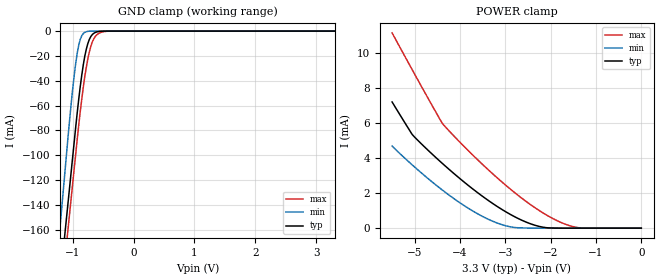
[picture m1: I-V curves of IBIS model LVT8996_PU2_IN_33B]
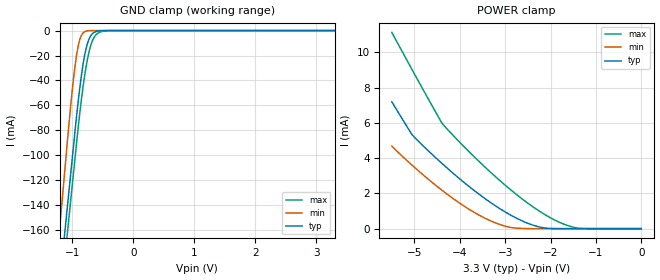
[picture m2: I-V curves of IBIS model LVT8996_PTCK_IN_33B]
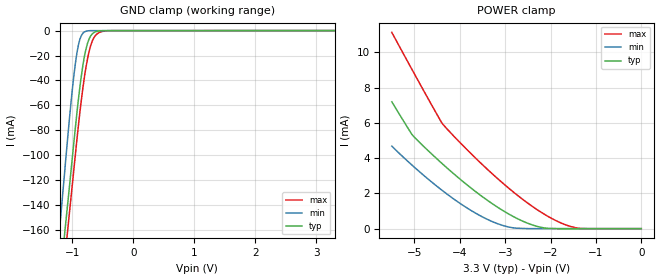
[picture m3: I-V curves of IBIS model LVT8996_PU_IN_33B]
| TEXAS INSTRUMENTS INCORPORATED
| Standard Linear and Logic Group
| IBIS Model of SN74LVT8996
| 3.3-V 10-BIT ADDRESSABLE SCAN PORTS
| This file contains package information for the following:
|  SOIC 24-pin (DW) package as [Component] IBIS_TOP_DW
| This device can be powered at the following Vccs:
|  3.3 volt Vcc
| This file provides unique models under the [Model Selector] for each Vcc.
| For operation at a specific Vcc, select the appropriate model after each
| [Model Selector] keyword.
[IBIS Ver]   3.2
[Comment char]  |_char
[File Name]   sn74lvt8996.ibs
[File Rev]   1.1 | x_die
[Date]   Apr 2, 2004
[Source]   Data created from TI-SPICE simulations at TI-SLL.
[Notes]   The following is an IBIS list for the IBIS_TOP.
   Please contact sllibis@ti.com with questions and
   comments concerning SLL IBIS models.
   NOTE:  The gnd_clamp, pwr_clamp, pullup, and pulldown data
   for ranges beyond GND-VCC may have modeling inaccuracies due
   to convergence problems over the extended IBIS ranges.
|   FILE REV HISTORY
|   1.1  Package R,L C data corrected.
[Disclaimer] Property of Texas Instruments Incorporated.  Unauthorized
   reproduction and/or distribution is strictly prohibited.
   This product is protected under copyright law.
   Created  2002, (C) Copyright  2002, Texas Instruments
   Incorporated, All Rights Reserved
   UNLESS THERE IS A SIGNED, WRITTEN AGREEMENT TO THE
   CONTRARY, TEXAS INSTRUMENTS (TI) IS PROVIDING THE IBIS
   MODELS  AND WITHOUT ANY WARRANTY, EXPRESSED OR
   IMPLIED.  TI assumes no liability for:
   1) the accuracy of the IBIS models provided to your
   company;
   2) the proper functioning of these IBIS Models in your
   design or for any resulting applications; or
   3) infringement of patents, copyrights or intellectual
   property rights resulting from your use of these IBIS
   models.
   TI provides IBIS Models as a service to our customers.
   You and your company shall not distribute, sell or give
   these models to anyone else without prior written
   permission from TI.
   TI reserves the right to make changes to our products or
   to discontinue any semiconductor product or service
   without notice, and advises our customers to obtain the
   latest version of relevant information to verify, before
   placing orders, that the information being relied on is
   current.
   Please be aware that your receipt and use of the IBIS
   information provided shall serve as acceptance of these
   terms and conditions.  If you do not accept these terms,
   you should return or destroy the IBIS models and any
   other accompanying information immediately.
| Component IBIS_TOP_DW 24-pin SOIC
[Component]   IBIS_TOP_DW
[Manufacturer]   Texas Instruments, Inc.
[Package]
|   typ   min   max
R_pkg   3.700e-02   3.000e-02   4.700e-02
L_pkg   5.146e-09   3.993e-09   6.885e-09
C_pkg   7.580e-13   5.120e-13   1.067e-12
[Pin]   signal_name   model_name   R_pin   L_pin   C_pin
1   A4   LVT8996_PU_IN   3.900e-02   6.885e-09   1.067e-12
2   A3   LVT8996_PU_IN   4.200e-02   5.950e-09   9.580e-13
3   A2   LVT8996_PU_IN   4.700e-02   5.317e-09   7.910e-13
4   A1   LVT8996_PU_IN   3.100e-02   4.651e-09   6.110e-13
5   A0   LVT8996_PU_IN   3.000e-02   3.993e-09   5.120e-13
6   NBYP   LVT8996_PU_IN   3.000e-02   4.083e-09   6.110e-13
7   GND   GND   3.000e-02   4.083e-09   6.110e-13
8   PTDO   LVT8996_TRI   3.000e-02   3.993e-09   5.120e-13
9   PTCK   LVT8996_PTCK_IN   3.100e-02   4.652e-09   6.110e-13
10   PTMS   LVT8996_PU2_IN   4.700e-02   5.317e-09   7.910e-13
11   PTDI   LVT8996_PU2_IN   4.200e-02   5.950e-09   9.590e-13
12   NPTRST   LVT8996_PU2_IN   3.900e-02   6.885e-09   1.067e-12
13   NSTRST   LVT8996_OUT   3.900e-02   6.885e-09   1.067e-12
14   STDO   LVT8996_TRI   4.200e-02   5.950e-09   9.590e-13
15   STMS   LVT8996_OUT   4.700e-02   5.317e-09   7.910e-13
16   STCK   LVT8996_OUT   3.100e-02   4.652e-09   6.110e-13
17   STDI   LVT8996_PU_IN   3.000e-02   3.993e-09   5.120e-13
18   NCON   LVT8996_OUT   3.000e-02   4.083e-09   6.100e-13
19   VCC   POWER   3.000e-02   4.083e-09   6.100e-13
20   A9   LVT8996_PU_IN   3.000e-02   3.993e-09   5.120e-13
21   A8   LVT8996_PU_IN   3.100e-02   4.651e-09   6.110e-13
22   A7   LVT8996_PU_IN   4.700e-02   5.317e-09   7.910e-13
23   A6   LVT8996_PU_IN   4.200e-02   5.950e-09   9.580e-13
24   A5   LVT8996_PU_IN   3.900e-02   6.885e-09   1.067e-12
| Component IBIS_TOP_PW 24-pin TSSOP
[Component]   IBIS_TOP_PW
[Manufacturer]   Texas Instruments, Inc.
[Package]
|   typ   min   max
R_pkg   3.900e-02   3.000e-02   4.600e-02
L_pkg   2.685e-09   2.367e-09   3.177e-09
C_pkg   3.200e-13   2.520e-13   4.340e-13
[Pin]   signal_name   model_name   R_pin   L_pin   C_pin
1		A4		LVT8996_PU_IN	3.70E-02	3.15E-09	4.34E-13
2		A3		LVT8996_PU_IN	3.40E-02	2.63E-09	3.41E-13
3		A2		LVT8996_PU_IN	3.20E-02	2.86E-09	3.47E-13
4		A1		LVT8996_PU_IN	4.20E-02	2.74E-09	2.90E-13
5		A0		LVT8996_PU_IN	4.60E-02	2.60E-09	2.62E-13
6		NBYP		LVT8996_PU_IN	4.30E-02	2.41E-09	2.66E-13
7		GND		GND			4.20E-02	2.37E-09	2.62E-13
8		PTDO		LVT8996_TRI		4.40E-02	2.46E-09	2.52E-13
9		PTCK		LVT8996_PTCK_IN	4.20E-02	2.54E-09	2.74E-13
10		PTMS		LVT8996_PU2_IN	3.00E-02	2.62E-09	3.32E-13
11		PTDI		LVT8996_PU2_IN	3.70E-02	2.67E-09	3.46E-13
12		NPTRST	LVT8996_PU2_IN	3.90E-02	3.18E-09	4.33E-13
13		NSTRST	LVT8996_OUT		3.70E-02	3.11E-09	4.31E-13
14		STDO		LVT8996_TRI		3.70E-02	2.66E-09	3.45E-13
15		STMS		LVT8996_OUT		3.10E-02	2.74E-09	3.40E-13
16		STCK		LVT8996_OUT		4.20E-02	2.65E-09	2.82E-13
17		STDI		LVT8996_PU_IN	4.60E-02	2.53E-09	2.57E-13
18		NCON		LVT8996_OUT		4.40E-02	2.43E-09	2.66E-13
19		VCC		POWER			4.40E-02	2.43E-09	2.66E-13
20		A9		LVT8996_PU_IN	4.60E-02	2.53E-09	2.57E-13
21		A8		LVT8996_PU_IN	4.20E-02	2.65E-09	2.82E-13
22		A7		LVT8996_PU_IN	3.10E-02	2.74E-09	3.39E-13
23		A6		LVT8996_PU_IN	3.60E-02	2.65E-09	3.44E-13
24		A5		LVT8996_PU_IN	3.70E-02	3.11E-09	4.31E-13
| Model LVT8996_PU2_IN
[Model Selector]   LVT8996_PU2_IN
LVT8996_PU2_IN_33B   3.3 volt Vcc
| Model LVT8996_PTCK_IN
[Model Selector]   LVT8996_PTCK_IN
LVT8996_PTCK_IN_33B   3.3 volt Vcc
| Model LVT8996_PU_IN
[Model Selector]   LVT8996_PU_IN
LVT8996_PU_IN_33B   3.3 volt Vcc
| Model LVT8996_OUT
[Model Selector]   LVT8996_OUT
LVT8996_OUT_33B   3.3 volt Vcc
| Model LVT8996_TRI
[Model Selector]   LVT8996_TRI
LVT8996_TRI_33B   3.3 volt Vcc
| Models and submodels in the file (5): LVT8996_PU2_IN_33B (Input), LVT8996_PTCK_IN_33B (Input), LVT8996_PU_IN_33B (Input), LVT8996_OUT_33B (Output), LVT8996_TRI_33B (3-state)
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[Model]   LVT8996_PU2_IN_33B
Model_type  Input
Vinl=0.8
Vinh=2.0
| variable   typ   min   max
C_comp   3.18pF   2.51pF   4.48pF
[Temperature Range]   40   -40   100
| Ambient temperature   25   -40   85
[Voltage range]   3.3   2.7   3.6
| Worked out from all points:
|   GND clamp passes 1 mA (typ) near -0.62 V on its own axis
|   POWER clamp passes 1 mA (typ) near -3.03 V on its own axis
[GND Clamp]
| LVT8996_PU2_IN_33B
|   Voltage   I(typ)   I(min)   I(max)
-5.5V     -2.287A    -2.545A    -2.286A
-1.23V    -213.2mA   -170.8mA   -233.6mA
-1.2V     -198.6mA   -154.2mA   -219.2mA
-1.13V    -164.7mA   -115.4mA   -185.6mA
-1.105V   -152.6mA   -101.6mA   -173.6mA
-1.075V   -138.1mA   -85mA      -159.2mA
-975mV    -89.69mA   -36mA      -111.2mA
-900mV    -54.93mA   -11.38mA   -75.88mA
-775mV    -14.5mA    -474.9uA   -29.04mA
-700mV    -4.254mA   -33.37uA   -12.08mA
-600mV    -616.1uA   -10.07uA   -2.838mA
3.3V      16.16pA    8.699pA    -7.502nA
[POWER Clamp]
| LVT8996_PU2_IN_33B
|   Voltage   I(typ)   I(min)   I(max)
-5.5V     7.191mA    4.679mA    11.13mA
-5.055V   5.335mA    3.603mA    9.023mA
-4.39V    3.688mA    2.171mA    5.968mA
-3.895V   2.595mA    1.261mA    4.615mA
-3.45V    1.713mA    598.2uA    3.501mA
-3.055V   1.033mA    183.2uA    2.585mA
-2.715V   547.5uA    22.73uA    1.862mA
-2.17V    55.3uA     4.611nA    869.2uA
-1.83V    1.773uA    15.23pA    391.7uA
-1.525V   8.75nA     13.18pA    99.72uA
-1.26V    93.03pA    11.89pA    5.075uA
-95.1fV   16.16pA    5.854pA    469.5pA
[Model]   LVT8996_PTCK_IN_33B
Model_type  Input
Vinl=0.8
Vinh=2.0
| variable   typ   min   max
C_comp   3.18pF   2.51pF   4.49pF
[Temperature Range]   40   -40   100
| Ambient temperature   25   -40   85
[Voltage range]   3.3   2.7   3.6
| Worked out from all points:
|   GND clamp passes 1 mA (typ) near -0.62 V on its own axis
|   POWER clamp passes 1 mA (typ) near -3.03 V on its own axis
[GND Clamp]
| LVT8996_PTCK_IN_33B
|   Voltage   I(typ)   I(min)   I(max)
-5.5V     -2.287A    -2.545A    -2.286A
-1.225V   -210.7mA   -168.1mA   -231.2mA
-1.195V   -196.2mA   -151.4mA   -216.8mA
-1.135V   -167.1mA   -118.2mA   -188mA
-1.105V   -152.6mA   -101.6mA   -173.6mA
-1.075V   -138.1mA   -84.99mA   -159.2mA
-975mV    -89.68mA   -35.99mA   -111.2mA
-900mV    -54.92mA   -11.37mA   -75.86mA
-775mV    -14.49mA   -464.5uA   -29.03mA
-700mV    -4.239mA   -23.21uA   -12.06mA
-600mV    -600.8uA   -202.5nA   -2.821mA
3.3V      16.16pA    8.099pA    391.9pA
[POWER Clamp]
| LVT8996_PTCK_IN_33B
|   Voltage   I(typ)   I(min)   I(max)
-5.5V     7.191mA    4.679mA    11.13mA
-5.055V   5.335mA    3.603mA    9.023mA
-4.39V    3.688mA    2.171mA    5.968mA
-3.895V   2.595mA    1.261mA    4.615mA
-3.45V    1.713mA    598.2uA    3.501mA
-3.055V   1.033mA    183.2uA    2.585mA
-2.715V   547.5uA    22.73uA    1.862mA
-2.17V    55.3uA     4.609nA    869.2uA
-1.83V    1.773uA    13.4pA     391.7uA
-1.525V   8.748nA    11.66pA    99.72uA
-1.26V    91.77pA    10.63pA    5.075uA
-95.1fV   16.16pA    5.854pA    469.5pA
[Model]   LVT8996_PU_IN_33B
Model_type  Input
Vinl=0.8
Vinh=2.0
| variable   typ   min   max
C_comp   3.17pF   2.51pF   4.59pF
[Temperature Range]   40   -40   100
| Ambient temperature   25   -40   85
[Voltage range]   3.3   2.7   3.6
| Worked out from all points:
|   GND clamp passes 1 mA (typ) near -0.62 V on its own axis
|   POWER clamp passes 1 mA (typ) near -3.03 V on its own axis
[GND Clamp]
| LVT8996_PU_IN_33B
|   Voltage   I(typ)   I(min)   I(max)
-5.5V     -2.287A    -2.545A    -2.286A
-1.225V   -210.7mA   -168.1mA   -231.2mA
-1.195V   -196.2mA   -151.5mA   -216.8mA
-1.13V    -164.7mA   -115.5mA   -185.6mA
-1.1V     -150.2mA   -98.85mA   -171.2mA
-1.075V   -138.1mA   -85.02mA   -159.2mA
-975mV    -89.72mA   -36.02mA   -111.3mA
-900mV    -54.96mA   -11.41mA   -75.91mA
-775mV    -14.53mA   -496.9uA   -29.08mA
-700mV    -4.283mA   -54.97uA   -12.11mA
-600mV    -648.6uA   -31.02uA   -2.874mA
3.3V      16.16pA    8.699pA    -7.703nA
[POWER Clamp]
| LVT8996_PU_IN_33B
|   Voltage   I(typ)   I(min)   I(max)
-5.5V     7.191mA    4.679mA    11.13mA
-5.055V   5.335mA    3.603mA    9.023mA
-4.39V    3.688mA    2.171mA    5.968mA
-3.895V   2.595mA    1.261mA    4.615mA
-3.45V    1.713mA    598.2uA    3.501mA
-3.055V   1.033mA    183.2uA    2.585mA
-2.715V   547.5uA    22.73uA    1.862mA
-2.17V    55.3uA     4.611nA    869.2uA
-1.83V    1.773uA    15.23pA    391.7uA
-1.525V   8.75nA     13.18pA    99.72uA
-1.26V    93.03pA    11.89pA    5.075uA
-95.1fV   16.16pA    5.854pA    469.5pA
